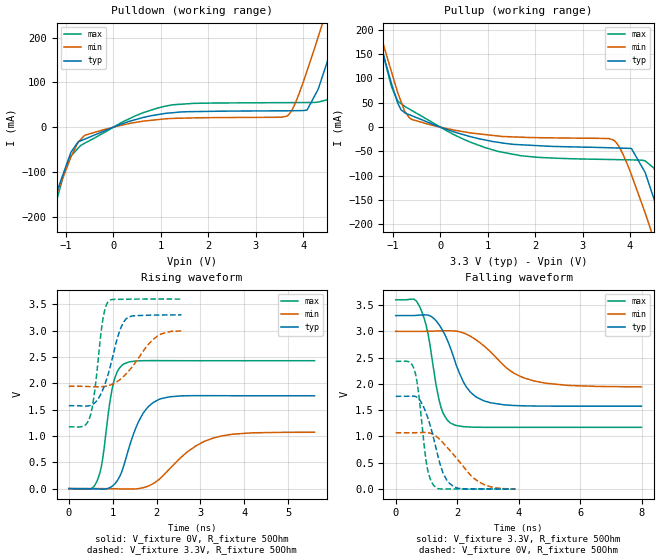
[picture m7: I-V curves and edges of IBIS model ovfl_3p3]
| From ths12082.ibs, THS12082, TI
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|   ovfl_3p3 Model
[Model]   ovfl_3p3
Model_type   Output
Polarity   Non-Inverting
Vmeas = 1.65
Vref = 1.65
Cref = 2pF
Rref = 50
|   typ   min   max
|   (nom PVT)   (fast PVT)   (slow PVT)
C_comp   1.924e-12   1.903e-12   2.001e-12
|ON state : BUFFER OUTPUT TURNED HIGH
|C_comp   1.924e-12   1.903e-12   2.001e-12
|OFF state: BUFFER OUTPUT TURNED LOW
|C_comp   1.784e-12   1.775e-12   1.813e-12
| Where nom  PVT is Nominal Process, 3.3V, 27C
|   Fast PVT is Strong Process,  3.6V, -55C
|   Slow PVT is Weak Process,   3V, 125C
[Voltage Range]   3.3   3   3.6
|Ambient Temperature   25   125   -55
|Junction Temperature
[Temperature Range]   27   125   -55
[Pullup Reference]   3.3   3   3.6
[Pulldown Reference]   0   0   0
[Power Clamp Reference]   3.3   3   3.6
[GND Clamp Reference]   0   0   0
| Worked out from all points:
|   slope of the pulldown table from 0 to 0.495 V, typ, clamps not added: 28 ohm
|   slope of the pullup table from 0 to 0.495 V, typ, clamps not added: 31.6 ohm
|   falling waveform, V_fixture 3.3V, R_fixture 50Ohm: 20-80 % time 743ps typ, 1.28ns min, 437ps max; typ from 3.3 V to 1.58 V
|   rising waveform, V_fixture 0V, R_fixture 50Ohm: 20-80 % time 461ps typ, 888ps min, 244ps max; typ from 0 V to 1.76 V
|   rising waveform, V_fixture 3.3V, R_fixture 50Ohm: 20-80 % time 348ps typ, 586ps min, 201ps max; typ from 1.58 V to 3.3 V
|   falling waveform, V_fixture 0V, R_fixture 50Ohm: 20-80 % time 500ps typ, 945ps min, 285ps max; typ from 1.76 V to 0 V
[Pulldown]
|   Voltage   I(typ)   I(min)   I(max)
-3.3V     -923.6mA   -847.5mA   -1.036A
-1.67V    -308.9mA   -293.9mA   -354.5mA
-1.372V   -205.5mA   -201.5mA   -230.4mA
-896.4mV  -56.13mA   -66.47mA   -64.48mA
-591mV    -26.14mA   -17.73mA   -34.96mA
1.098V    30.73mA    18.6mA     46.91mA
3.66V     36.44mA    24.72mA    54.7mA
4.082V    38.22mA    125.7mA    54.91mA
4.468V    133mA      252.2mA    60.08mA
4.662V    201.8mA    318.6mA    95.82mA
5.062V    345.8mA    460.1mA    239.3mA
6.6V      931.7mA    1.025A     847.3mA
[Pullup]
|   Voltage   I(typ)   I(min)   I(max)
-3.3V     970.9mA    949.6mA    1.007A
-1.325V   196.3mA    214.4mA    194.4mA
-1.03V    89.27mA    113.7mA    83.04mA
-896.4mV  48.97mA    70.33mA    53.32mA
-591mV    23.07mA    15.51mA    33.59mA
1.246V    -31.57mA   -18.54mA   -50.45mA
3.645V    -42.63mA   -26.12mA   -66.6mA
4.033V    -44.37mA   -98.86mA   -67.28mA
4.468V    -136.4mA   -219.7mA   -81.29mA
4.691V    -208.1mA   -289.2mA   -134.2mA
4.871V    -266.7mA   -346.1mA   -198.4mA
6.6V      -907.1mA   -928.5mA   -902.6mA
[Ramp]
R_load = 50
|   typ   min   max
dV/dt_r   1.05827/4.5886e-10   0.64206/8.80392e-10   1.4574/2.43062e-10
dV/dt_f   1.03452/7.39493e-10   0.633873/1.27526e-09   1.45583/4.3646e-10
[Falling Waveform]
V_fixture = 3.3V
V_fixture_min = 3V
V_fixture_max = 3.6V
R_fixture = 50Ohm
|   Time   V(typ)   V(min)   V(max)
0s        3.3V       3V         3.6V
786ps     3.31V      3V         3.464V
1.058ns   3.308V     3.001V     2.936V
1.444ns   3.098V     3.008V     1.62V
1.796ns   2.661V     3.01V      1.251V
2.304ns   1.937V     2.946V     1.184V
2.918ns   1.669V     2.7V       1.174V
3.69ns    1.595V     2.267V     1.174V
4.472ns   1.58V      2.062V     1.174V
7.998ns   1.576V     1.944V     1.174V
[Rising Waveform]
V_fixture = 0V
V_fixture_min = 0V
V_fixture_max = 0V
R_fixture = 50Ohm
|   Time   V(typ)   V(min)   V(max)
0s        1.442nV    2.279nV    1.191nV
488ps     -2.054mV   268.7uV    -9.221mV
642ps     -6.708mV   90.59uV    141.3mV
762ps     -10.57mV   -549.1uV   514.2mV
1.004ns   55.97mV    -3.067mV   1.96V
1.242ns   409mV      -6.677mV   2.362V
1.688ns   1.424V     15.7mV     2.429V
2.096ns   1.707V     203.6mV    2.431V
3.29ns    1.765V     960mV      2.429V
5.6ns     1.764V     1.07V      2.429V
[Rising Waveform]
V_fixture = 3.3V
V_fixture_min = 3V
V_fixture_max = 3.6V
R_fixture = 50Ohm
|   Time   V(typ)   V(min)   V(max)
0s        1.576V     1.943V     1.174V
334ps     1.568V     1.942V     1.185V
480ps     1.577V     1.937V     1.36V
588ps     1.627V     1.934V     1.843V
762ps     1.852V     1.937V     3.139V
894ps     2.166V     1.955V     3.546V
1.136ns   2.938V     2.051V     3.595V
1.304ns   3.224V     2.177V     3.597V
2.016ns   3.296V     2.896V     3.6V
2.566ns   3.3V       2.993V     3.6V
[Falling Waveform]
V_fixture = 0V
V_fixture_min = 0V
V_fixture_max = 0V
R_fixture = 50Ohm
|   Time   V(typ)   V(min)   V(max)
0s        1.764V     1.07V      2.429V
426ps     1.766V     1.07V      2.424V
612ps     1.764V     1.071V     2.26V
736ps     1.726V     1.073V     1.863V
1.006ns   1.419V     1.075V     474.5mV
1.252ns   922.6mV    1.03V      58.43mV
1.542ns   305mV      878.1mV    -3.172mV
1.884ns   45.49mV    652.9mV    484.5uV
2.69ns    1.306mV    141.3mV    113.3uV
3.894ns   185.4uV    2.286mV    123.1uV
